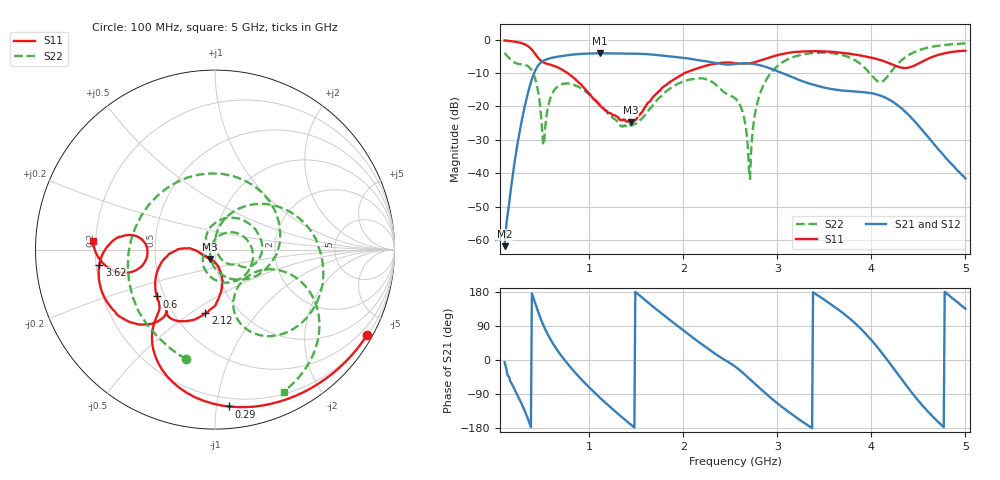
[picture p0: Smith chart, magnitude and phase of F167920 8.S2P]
!  2-Port S-parameters saved by WinCal
! VAR MeasName=S-Parameters (CALIBRATED_DATA) read from VNA (N5242A)
! VAR MeasDate=2016-11-22 9:53:53
! VAR NAME=F167920 8
! VAR FILENAME=F167920 8.S2P
! VAR DATE=2016-11-22 9:53:53
! VAR PHYS_PORTS=1,2
# Hz S DB R 50
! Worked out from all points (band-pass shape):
!   491 points, 100 MHz to 5 GHz, reference 50 ohm
!   highest |S21| = -4.09 dB at 1.11 GHz (marker M1); lowest = -61.8 dB at 100 MHz (marker M2)
!   |S21| within 3 dB of the highest: 476.9 MHz to 2.364 GHz (1.887 GHz wide, 133 % of centre); 2.627 GHz to 2.682 GHz (55.21 MHz wide, 2.08 % of centre)
!   lowest |S11| = -24.7 dB at 1.44 GHz (marker M3), VSWR 1.12, Z = 47.1 - j4.87 ohm
!   |S11| at or under -10 dB: 768.9 MHz to 2.014 GHz (1.245 GHz wide, 89.5 % of centre)
!   |S22| runs from -41.7 to -1.1 dB; largest |S21 - S12| = 0.0016
!   S11 on the Smith chart (normalised r, x): 100 MHz: 0.22, -3.82; 290 MHz: 0.14, -1.08; 600 MHz: 0.45, -0.29; 2.12 GHz: 0.70, -0.57; 3.62 GHz: 0.21, -0.06; 5 GHz: 0.19, +0.04
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1e8  -0.25 -29.3  -61.81 -6.0  -62.98 4.7  -3.97 -104.7
1.8e8  -0.50 -52.2  -41.93 -65.0  -42.05 -65.7  -6.34 -178.0
2.9e8  -1.14 -85.0  -23.18 -120.7  -23.18 -120.5  -7.45 84.8
4.2e8  -4.09 -124.1  -9.63 153.8  -9.62 153.8  -11.25 -32.2
5.1e8  -6.78 -132.7  -6.37 93.1  -6.36 93.1  -31.57 -170.0
6e8  -7.62 -141.1  -5.45 49.2  -5.45 49.2  -16.49 38.6
9.2e8  -13.59 179.8  -4.23 -51.9  -4.23 -51.9  -14.70 -80.3
1.11e9  -19.61 -177.4  -4.09 -98.8  -4.08 -98.8  -19.36 -127.5
1.44e9  -24.70 -117.8  -4.20 -169.8  -4.20 -169.8  -25.68 163.5
1.74e9  -15.44 -76.5  -4.66 128.7  -4.66 128.6  -17.55 98.4
2.12e9  -8.89 -98.6  -5.97 55.5  -5.95 55.5  -11.74 16.1
2.55e9  -7.02 -127.4  -7.29 -17.0  -7.27 -17.0  -17.55 -38.6
2.64e9  -7.22 -128.4  -7.07 -35.2  -7.06 -35.2  -22.62 -54.7
2.71e9  -7.05 -127.6  -7.15 -50.9  -7.13 -50.9  -41.69 51.3
2.77e9  -6.67 -127.3  -7.39 -64.6  -7.37 -64.6  -21.09 84.6
2.88e9  -5.69 -129.0  -8.18 -89.0  -8.16 -89.2  -12.14 62.2
3.37e9  -3.46 -158.3  -13.40 -179.8  -13.37 180.0  -4.02 -18.1
3.62e9  -3.74 -172.5  -14.97 138.3  -14.98 138.1  -4.20 -46.8
3.95e9  -5.12 173.6  -15.85 66.3  -15.84 66.0  -9.00 -72.7
4.19e9  -7.06 170.3  -17.96 -6.6  -17.97 -6.9  -10.36 -21.5
4.51e9  -7.03 -165.7  -26.05 -110.4  -26.07 -110.8  -3.13 -33.7
5e9  -3.32 175.8  -41.57 135.2  -41.36 134.3  -1.13 -64.2
